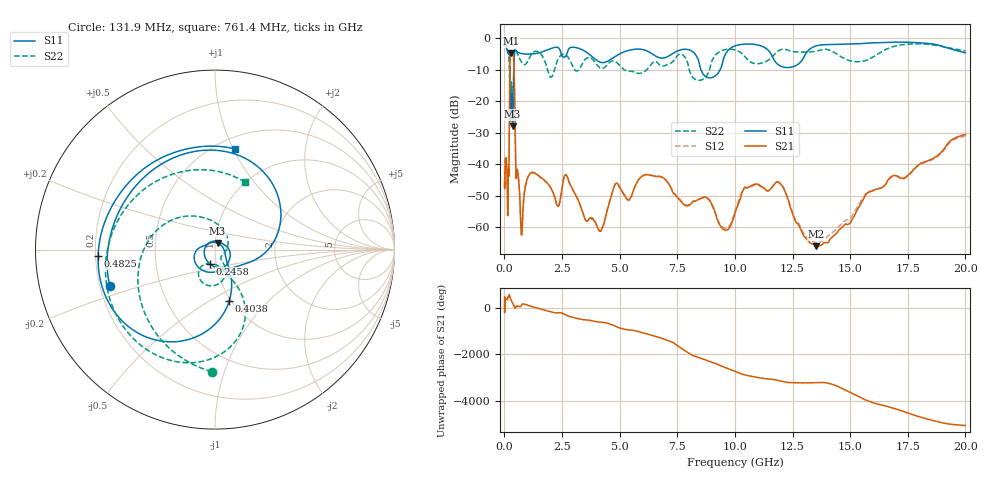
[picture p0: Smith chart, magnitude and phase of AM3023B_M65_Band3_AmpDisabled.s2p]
!Agilent Technologies,E8364B,MY43040894,A.07.50.67
!Agilent E8364B: A.07.50.67
!Date: Tuesday, October 27, 2020 10:48:56
!Correction: S11(Full 2 Port(1,2))
!S21(Full 2 Port(1,2))
!S12(Full 2 Port(1,2))
!S22(Full 2 Port(1,2))
!S2P File: Measurements: S11, S21, S12, S22:Log Frequency Sweep
# Hz S  dB  R 50
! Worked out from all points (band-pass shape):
!   3201 points, 10 MHz to 20 GHz, reference 50 ohm
!   highest |S21| = -4.74 dB at 288.2 MHz (marker M1); lowest = -66.1 dB at 13.52 GHz (marker M2)
!   |S21| within 3 dB of the highest: 240 MHz to 410.9 MHz (170.9 MHz wide, 52.5 % of centre)
!   lowest |S11| = -28.0 dB at 356.9 MHz (marker M3), VSWR 1.08, Z = 51.3 + j3.83 ohm
!   |S11| at or under -10 dB: 233.6 MHz to 405.7 MHz (172 MHz wide, 53.8 % of centre); 8.527 GHz to 9.357 GHz (829.8 MHz wide, 9.28 % of centre)
!   |S22| runs from -25.9 to -0.9 dB; largest |S21 - S12| = 0.012
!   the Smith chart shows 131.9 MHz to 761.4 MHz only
!   S11 on the Smith chart (normalised r, x): 131.9 MHz: 0.24, -0.16; 245.8 MHz: 0.93, -0.15; 403.8 MHz: 0.98, -0.61; 482.5 MHz: 0.21, -0.03; 761.4 MHz: 0.61, +1.02
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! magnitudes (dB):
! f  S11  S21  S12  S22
! 10 MHz  -0.6  -46.0  -41.8  -0.9
! 35.55 MHz  -1.3  -40.5  -40.2  -1.2
! 126.1 MHz  -4.0  -46.8  -46.5  -3.2
! 131.9 MHz  -4.1  -50.3  -49.7  -3.4
! 196.1 MHz  -5.0  -42.9  -42.9  -6.5
! 245.8 MHz  -21.5  -6.4  -6.4  -24.8
! 288.2 MHz  -18.6  -4.7  -4.8  -14.5
! 356.9 MHz  -28.0  -5.0  -5.0  -21.4
! 403.8 MHz  -10.6  -6.6  -6.7  -12.7
! 447.2 MHz  -3.7  -19.5  -19.5  -3.9
! 482.5 MHz  -3.7  -38.0  -38.1  -3.5
! 761.4 MHz  -4.9  -61.9  -61.9  -7.7
! 981.7 MHz  -5.0  -45.0  -45.0  -7.6
! 1.59 GHz  -4.4  -44.3  -44.4  -5.0
! 2.319 GHz  -2.9  -53.4  -53.5  -6.8
! 2.688 GHz  -5.4  -43.5  -43.5  -5.4
! 4.131 GHz  -7.5  -61.4  -61.3  -9.3
! 5.639 GHz  -3.5  -47.6  -47.6  -10.7
! 9.577 GHz  -5.2  -61.0  -60.4  -3.6
! 11.75 GHz  -7.4  -46.0  -45.9  -4.8
! 13.52 GHz  -2.4  -66.1  -65.1  -4.1
! 20 GHz  -4.6  -30.6  -31.0  -4.0
